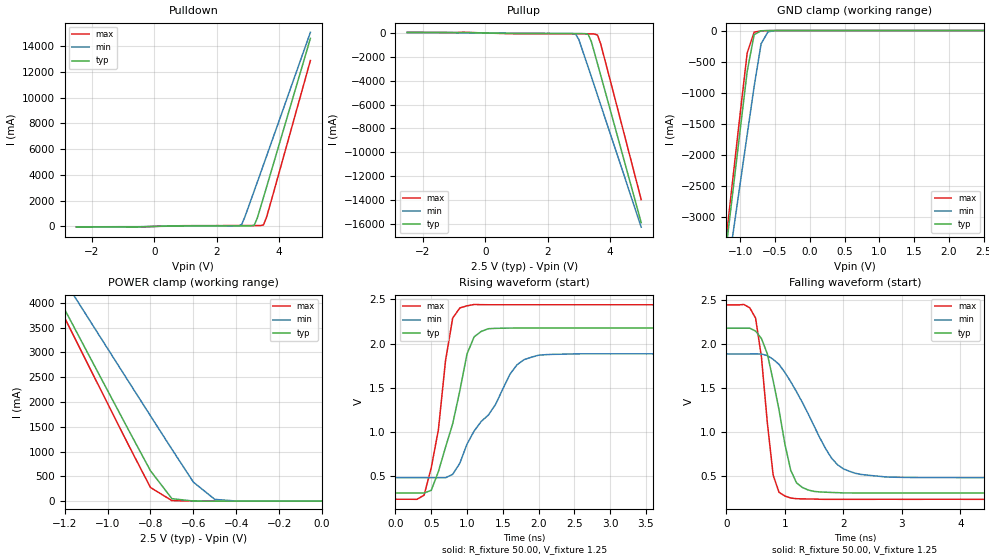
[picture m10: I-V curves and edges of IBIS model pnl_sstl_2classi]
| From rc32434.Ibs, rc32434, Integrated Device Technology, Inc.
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[Model]   pnl_sstl_2classi
Model_type   I/O
Polarity   Non-Inverting
Enable   Active-High
Vinl =  1.070V
Vinh =  1.430V
Vmeas =  1.250V
C_comp   0.40pF   0.30pF   0.50pF
[Temperature Range]   25.00   0.12k   0.000
[Voltage Range]   2.50V   2.25V   2.75V
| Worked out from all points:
|   slope of the pulldown table from 0 to 0.375 V, typ, clamps not added: 16.7 ohm
|   slope of the pullup table from 0 to 0.375 V, typ, clamps not added: 17.9 ohm
|   GND clamp passes 1 mA (typ) near -0.61 V on its own axis
|   POWER clamp passes 1 mA (typ) near -0.55 V on its own axis
|   rising waveform, R_fixture 50.00, V_fixture 1.25: 20-80 % time 333ps typ, 617ps min, 220ps max; typ from 0.302 V to 2.18 V
|   falling waveform, R_fixture 50.00, V_fixture 1.25: 20-80 % time 334ps typ, 675ps min, 206ps max; typ from 2.18 V to 0.302 V
[Pulldown]
| voltage   I(typ)   I(min)   I(max)
-2.5V     -39.06mA   -30.69mA   -45.06mA
-700mV    -41.12mA   -22.99mA   -57.56mA
800mV     36.53mA    21mA       50.82mA
2.7V      43.8mA     33.55mA    63.05mA
2.8V      43.87mA    157mA      63.15mA
2.9V      43.96mA    739mA      63.25mA
3.2V      93.74mA    2.764A     63.85mA
3.3V      658mA      3.445A     64.88mA
3.5V      2.276A     4.809A     121mA
3.6V      3.094A     5.493A     752mA
5V        14.61A     15.08A     12.89A
[Pullup]
| voltage   I(typ)   I(min)   I(max)
-2.5V     46.28mA    36.8mA     52.93mA
2.8V      -49.59mA   -32.78mA   -74.03mA
2.9V      -49.68mA   -97.84mA   -74.18mA
3V        -49.83mA   -545mA     -74.32mA
3.3V      -117mA     -2.873A    -75.53mA
3.4V      -707mA     -3.657A    -78.14mA
3.6V      -2.583A    -5.228A    -176mA
3.7V      -3.529A    -6.015A    -907mA
5V        -15.9A     -16.28A    -13.97A
[GND_clamp]
| voltage   I(typ)   I(min)   I(max)
-2.5V     -15.85A    -14.27A    -16.42A
-1.2V     -3.479A    -4.021A    -3.324A
-1.1V     -2.533A    -3.236A    -2.323A
-1V       -1.591A    -2.454A    -1.327A
-900mV    -657mA     -1.673A    -360mA
-800mV    -67.52mA   -898mA     -26.19mA
-700mV    -4.03mA    -212mA     -5.545mA
-600mV    -573uA     -19.82mA   -1.86mA
-400mV    -5.043uA   -60.46uA   -28.07uA
2.5V      22.05pA    22.8uA     -254pA
[POWER_clamp]
| voltage   I(typ)   I(min)   I(max)
-2.5V     14.55A     13.34A     14.99A
-1.3V     4.687A     5.125A     4.563A
-1.2V     3.868A     4.442A     3.697A
-1.1V     3.049A     3.76A      2.832A
-900mV    1.418A     2.399A     1.112A
-800mV    613mA      1.721A     275mA
-700mV    49.54mA    1.047A     10.44mA
-600mV    1.81mA     384mA      1.901mA
-500mV    183uA      34.74mA    577uA
-400mV    16.57uA    1.896mA    79.12uA
0V        22.05pA    457pA      -591pA
[Ramp]
| variable   typ   min   max
dV/dt_r   1.05/0.24n   0.74/0.44n   1.28/0.17n
dV/dt_f   1.06/0.39n   0.70/0.62n   1.29/0.26n
R_load = 50.00
[Rising Waveform]
R_fixture = 50.00
V_fixture = 1.25
| time   V(typ)   V(min)   V(max)
0s        302mV      476mV      231mV
400ps     302mV      476mV      277mV
600ps     545mV      475mV      1.02V
700ps     822mV      475mV      1.807V
800ps     1.089V     514mV      2.289V
1ns       1.881V     857mV      2.428V
1.3ns     2.168V     1.188V     2.44V
1.7ns     2.176V     1.759V     2.44V
2ns       2.176V     1.867V     2.44V
9.9ns     2.176V     1.883V     2.44V
[Falling Waveform]
R_fixture = 50.00
V_fixture = 1.25
| time   V(typ)   V(min)   V(max)
0s        2.176V     1.883V     2.44V
500ps     2.143V     1.884V     2.291V
600ps     2.059V     1.882V     1.85V
800ps     1.581V     1.822V     507mV
900ps     1.25V      1.765V     310mV
1.1ns     562mV      1.568V     245mV
1.3ns     365mV      1.331V     235mV
1.8ns     308mV      697mV      230mV
2.3ns     302mV      513mV      230mV
9.9ns     302mV      476mV      231mV
